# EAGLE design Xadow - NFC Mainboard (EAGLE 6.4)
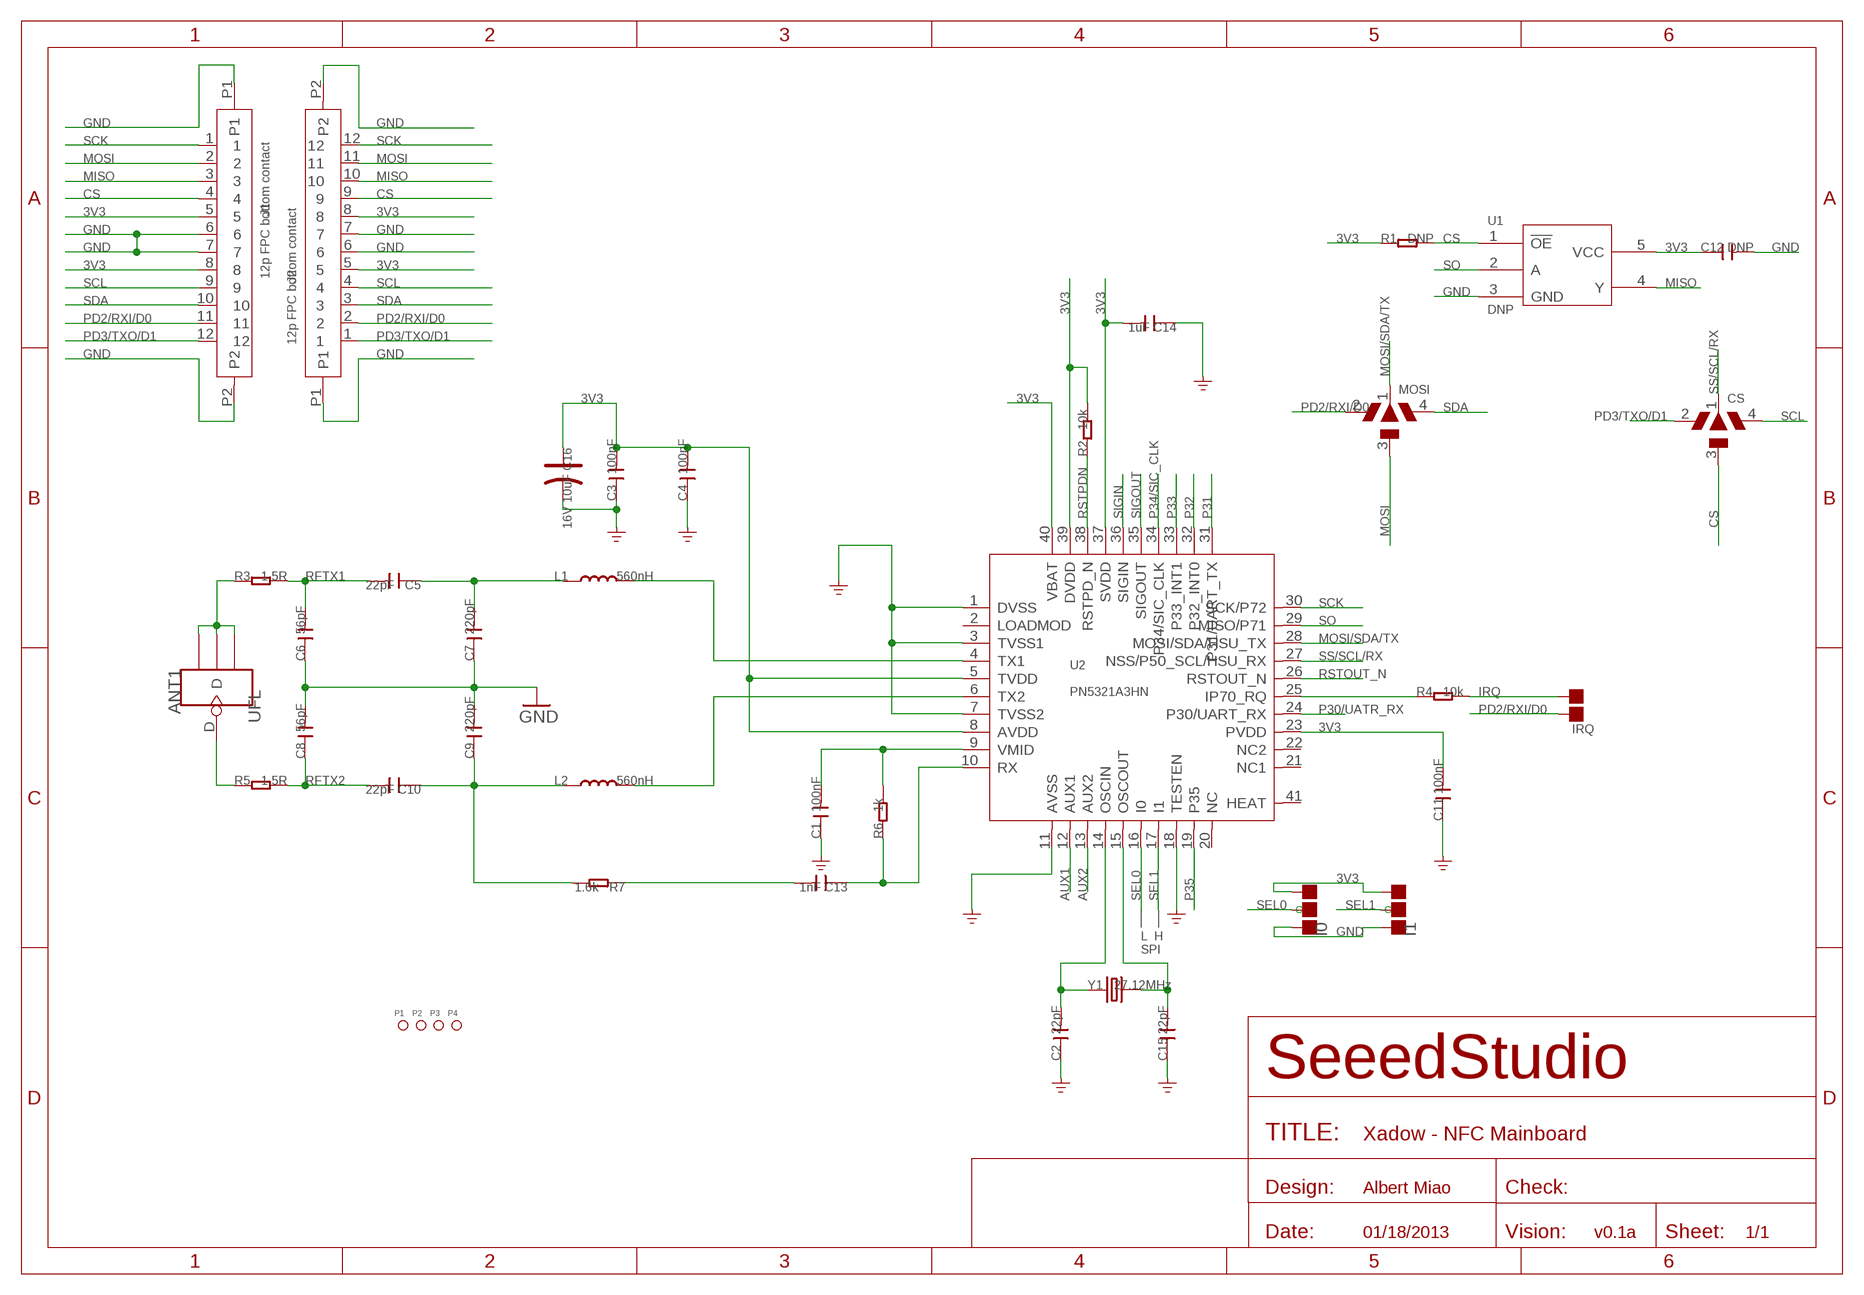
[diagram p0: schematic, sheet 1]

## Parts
ANT1  UFL  ANTENNA-U-FL  [4P-U-FL]
C1  100nF  C-0402  [C0402]
C2  22pF  C-0402  [C0402]
C3  100nF  C-0402  [C0402]
C4  100nF  C-0402  [C0402]
C5  22pF  C-0402  [C0402]
C6  56pF  C-0402  [C0402]
C7  220pF  C-0402  [C0402]
C8  56pF  C-0402  [C0402]
C9  220pF  C-0402  [C0402]
C10  22pF  C-0402  [C0402]
C11  100nF  C-0402  [C0402]
C12  DNP  C-0402  [C0402]
C13  1nF  C-0402  [C0402]
C14  1uF  C-0603  [C0603]
C15  22pF  C-0402  [C0402]
C16  16V 10uF  CAP-AVX-A  [AVX-A]
CS  DNP  PAD-JUMPER-4P  [4P-TRIANGLE]
I0  DNP  PAD-JUMPER-3P-40*40  [3P-SMD-4.1X1.5]
I1  DNP  PAD-JUMPER-3P-40*40  [3P-SMD-4.1X1.5]
IRQ  DNP  PAD-JUMPER-2P  [2P-SMD-1.78X1.27]
J1  12p FPC bottom contact  FPC052002-12LT  [12P-0.5]
J2  12p FPC bottom contact  FPC052002-12LT  [12P-0.5]
L1  560nH  L'0603'  [L0603]
L2  560nH  L'0603'  [L0603]
MOSI  DNP  PAD-JUMPER-4P  [4P-TRIANGLE]
P1  PAD-MARK  [ROUND-MARK-1.0]
P2  PAD-MARK  [ROUND-MARK-1.0]
P3  PAD-MARK  [ROUND-MARK-1.0]
P4  PAD-MARK  [ROUND-MARK-1.0]
R1  DNP  R-0402  [R0402]
R2  10k  R-0402  [R0402]
R3  1.5R  R-0402  [R0402]
R4  10k  R-0402  [R0402]
R5  1.5R  R-0402  [R0402]
R6  1k  R-0402  [R0402]
R7  1.6k  R-0402  [R0402]
U1  DNP  SN74LVC1G125DCKR  [SOT353]
U2  PN5321A3HN  PN532-HVQFN40  [HVQFN40]
Y1  27.12MHz  CRYSTAL'3225'  [4P-SMD-3.2X2.5]

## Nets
3V3: C3.2 C4.2 C11.2 C12.1 C14.2 C16.+ I0.00(L) I1.00(L) J1.5 J1.8 J2.5 J2.8 R1.1 R2.2 U1.5(VCC) U2.5(TVDD) U2.8(AVDD) U2.23(PVDD) U2.37(SVDD) U2.39(DVDD) U2.40(VBAT)
AUX1: U2.12(AUX1)
AUX2: U2.13(AUX2)
CS: CS.3 J1.4 J2.9 R1.2 U1.1(!OE!)
GND: C1.1 C2.1 C3.1 C4.1 C6.1 C7.1 C8.2 C9.2 C11.1 C12.2 C14.1 C15.1 C16.- I0.11(R) I1.11(R) J1.6 J1.7 J1.P1 J1.P2 J2.6 J2.7 J2.P1 J2.P2 U1.3(GND) U2.1(DVSS) U2.3(TVSS1) U2.7(TVSS2) U2.11(AVSS) U2.18(TESTEN)
IRQ: IRQ.1 R4.2
MISO: J1.3 J2.10 U1.4(Y)
MOSI: J1.2 J2.11 MOSI.3
MOSI/SDA/TX: MOSI.1 U2.28(MOSI/SDA/HSU_TX)
N$1: C2.2 U2.14(OSCIN) Y1.2
N$2: C15.2 U2.15(OSCOUT) Y1.4
N$3: L2.2 U2.6(TX2)
N$4: L1.2 U2.4(TX1)
N$5: C5.1 C7.2 L1.1
N$6: C13.2 R7.1
N$7: C9.1 C10.1 L2.1 R7.2
N$9: C1.2 R6.2 U2.9(VMID)
N$11: C13.1 R6.1 U2.10(RX)
N$15: R4.1 U2.25(IP70_RQ)
N$17: ANT1.D R5.1
N$18: ANT1.GND1 ANT1.GND2 ANT1.GND3 R3.1
P30/UATR_RX: U2.24(P30/UART_RX)
P31: U2.31(P31/UART_TX)
P32: U2.32(P32_INT0)
P33: U2.33(P33_INT1)
P34/SIC_CLK: U2.34(P34/SIC_CLK)
P35: U2.19(P35)
PD2/RXI/D0: IRQ.2 J1.11 J2.2 MOSI.2
PD3/TXO/D1: CS.2 J1.12 J2.1
RFTX1: C5.2 C6.2 R3.2
RFTX2: C8.1 C10.2 R5.2
RSTOUT_N: U2.26(RSTOUT_N)
RSTPDN: R2.1 U2.38(RSTPD_N)
SCK: J1.1 J2.12 U2.30(SCK/P72)
SCL: CS.4 J1.9 J2.4
SDA: J1.10 J2.3 MOSI.4
SEL0: I0.MM(C) U2.16(I0)
SEL1: I1.MM(C) U2.17(I1)
SIGIN: U2.36(SIGIN)
SIGOUT: U2.35(SIGOUT)
SO: U1.2(A) U2.29(MISO/P71)
SS/SCL/RX: CS.1 U2.27(NSS/P50_SCL/HSU_RX)
Unconnected: U2.2(LOADMOD) U2.20(NC) U2.21(NC1) U2.22(NC2) U2.41(HEAT)

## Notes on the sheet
- L | H
- SPI
- Albert Miao
- 01/18/2013 | v0.1a

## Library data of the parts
ANT1 = Connector:ANTENNA-U-FL
C1-C15 = Discrete:C*: Ceramic Capacitors
C16 = Discrete:CAP*: Electrolytic Capacitors,Tantalum Capacitors and Super Capacitors
CS MOSI = Discrete:PAD-JUMPER-4P
I0 I1 = Discrete:PAD-JUMPER-3P; PARTNO: DNP
IRQ = Discrete:PAD-JUMPER-2P; PARTNO: DNP
J1 J2 = template:FPC052002-12LT
L1 L2 = Discrete:L*
P1-P4 = Discrete:PAD-MARK; PARTNO: DNP
R1-R7 = Discrete:R*
U1 = Test:SN74LVC1G125DCKR: Signal bus buffer gate
U2 = IC:PN532: NFC Controller http://www.adafruit.com/datasheets/pn532ds.pdf
Y1 = Discrete:CRYSTAL*: CRYSTAL

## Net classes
0 default: width 0.152 mm, drill 0.305 mm, clearance 0.152 mm
1 GND: width 0.152 mm, drill 0.305 mm, clearance 0.152 mm to class 0, clearance 0.152 mm
3 usbvcc: width 0.203 mm, drill 0.305 mm, clearance 0.203 mm

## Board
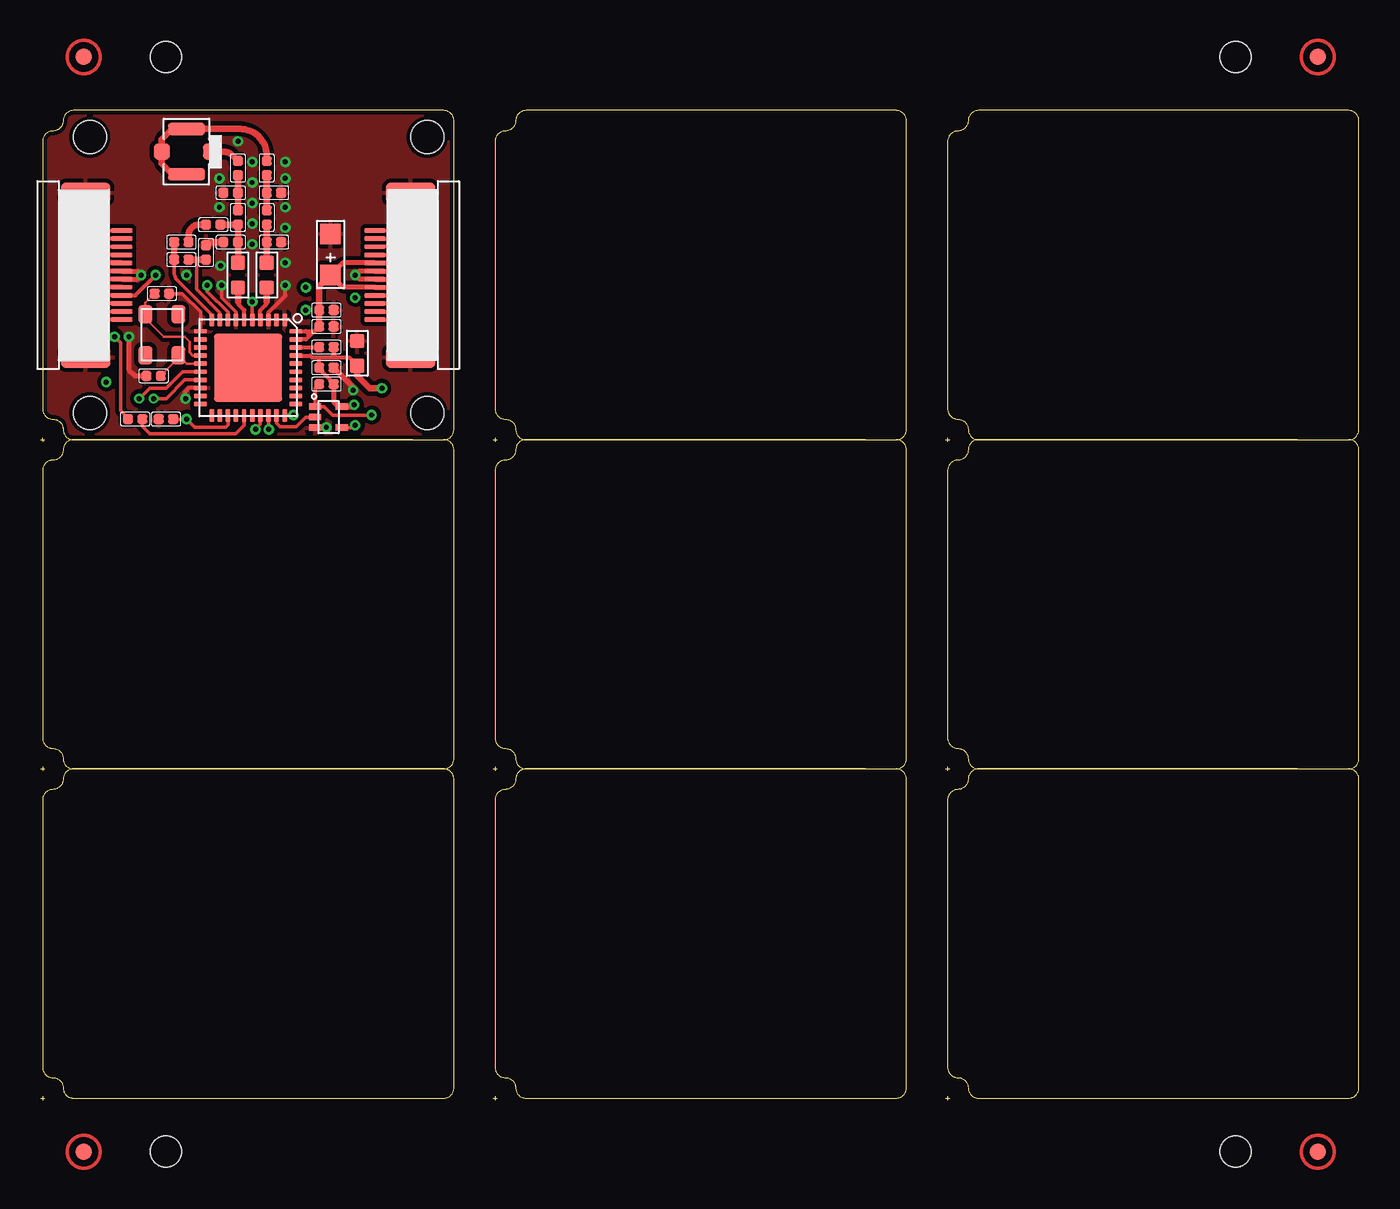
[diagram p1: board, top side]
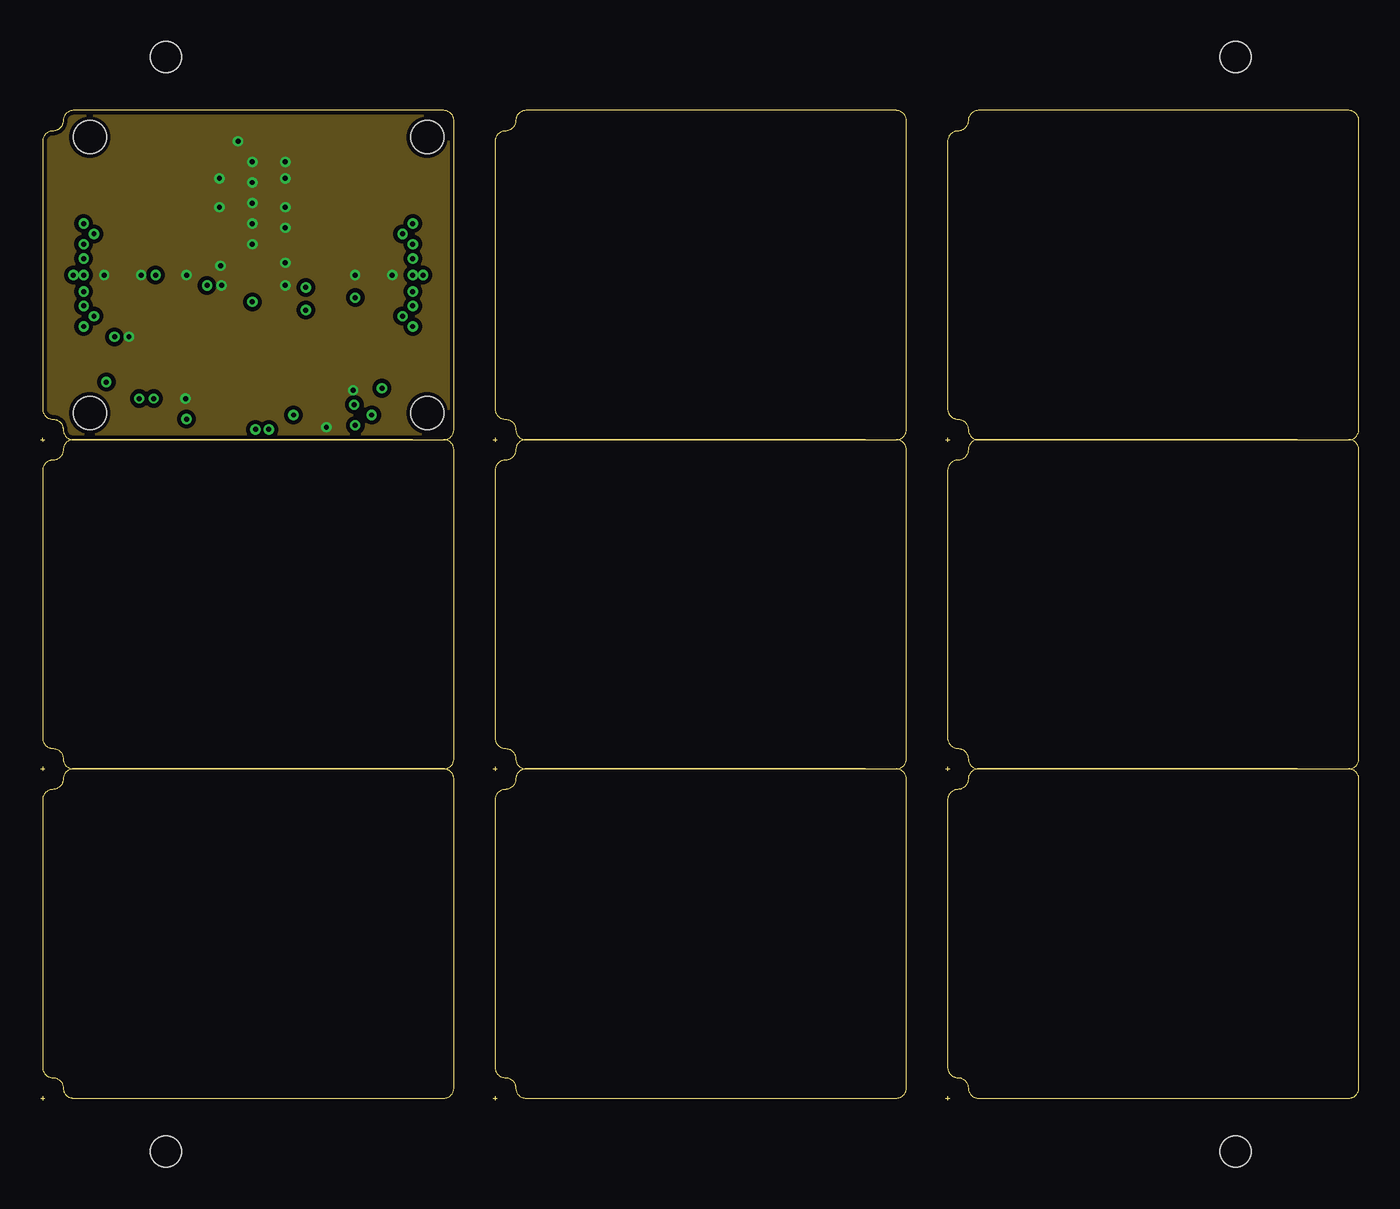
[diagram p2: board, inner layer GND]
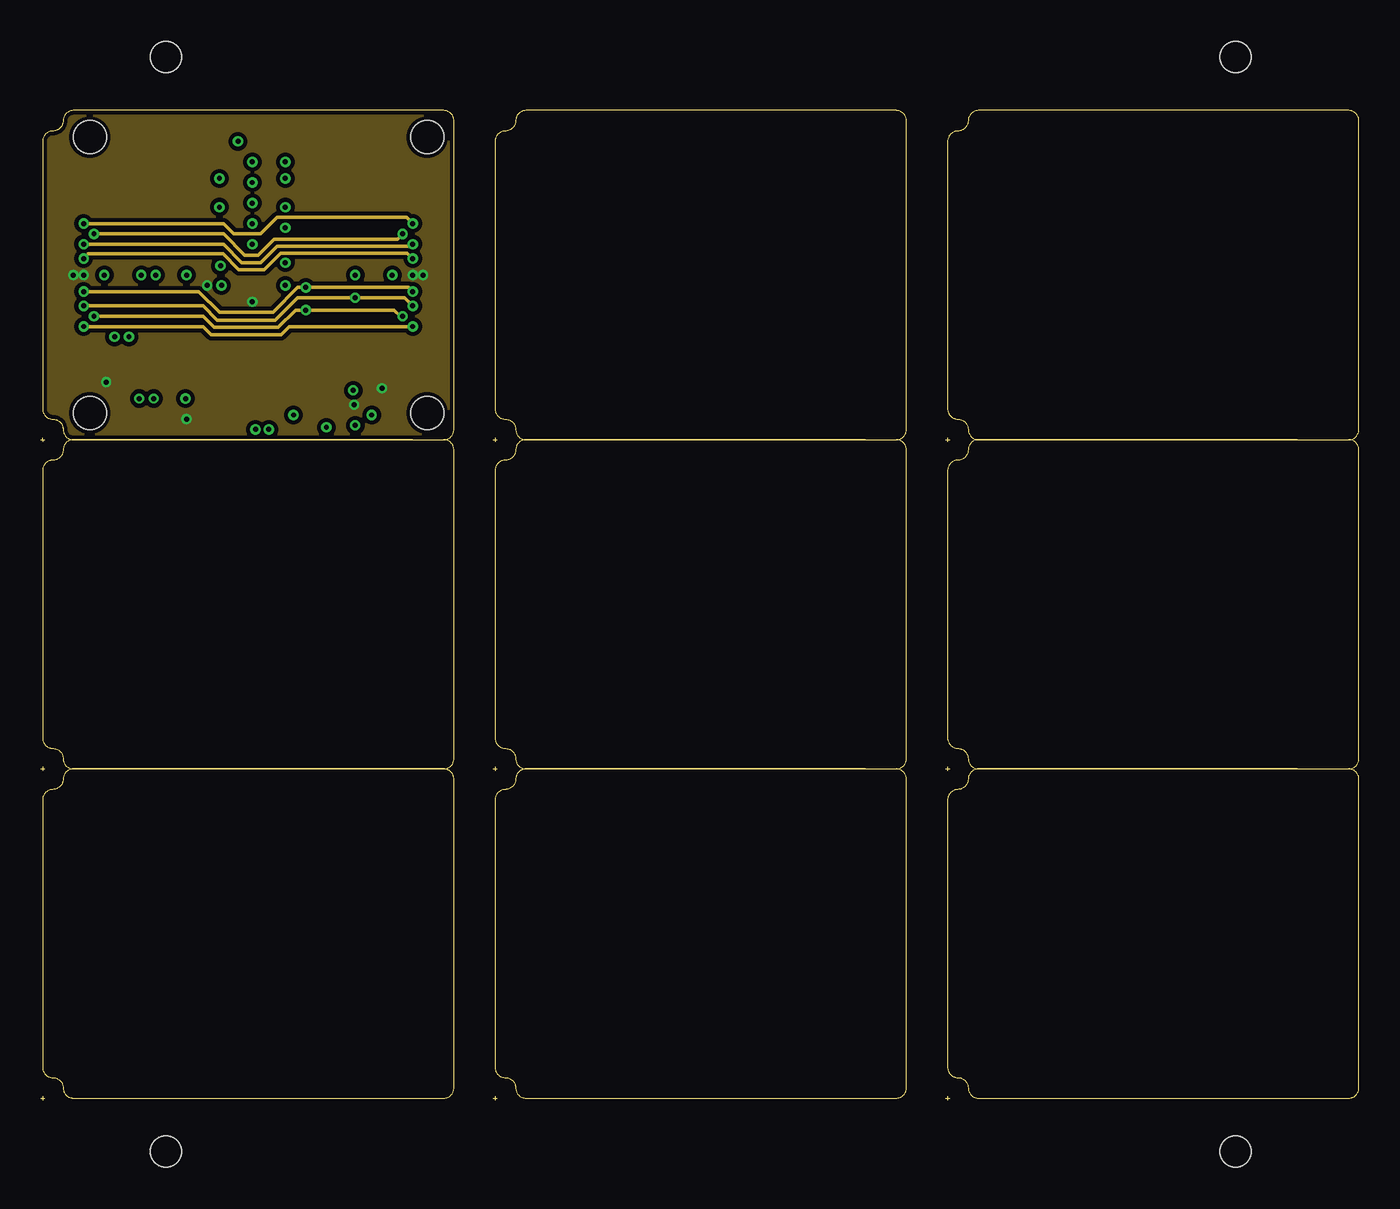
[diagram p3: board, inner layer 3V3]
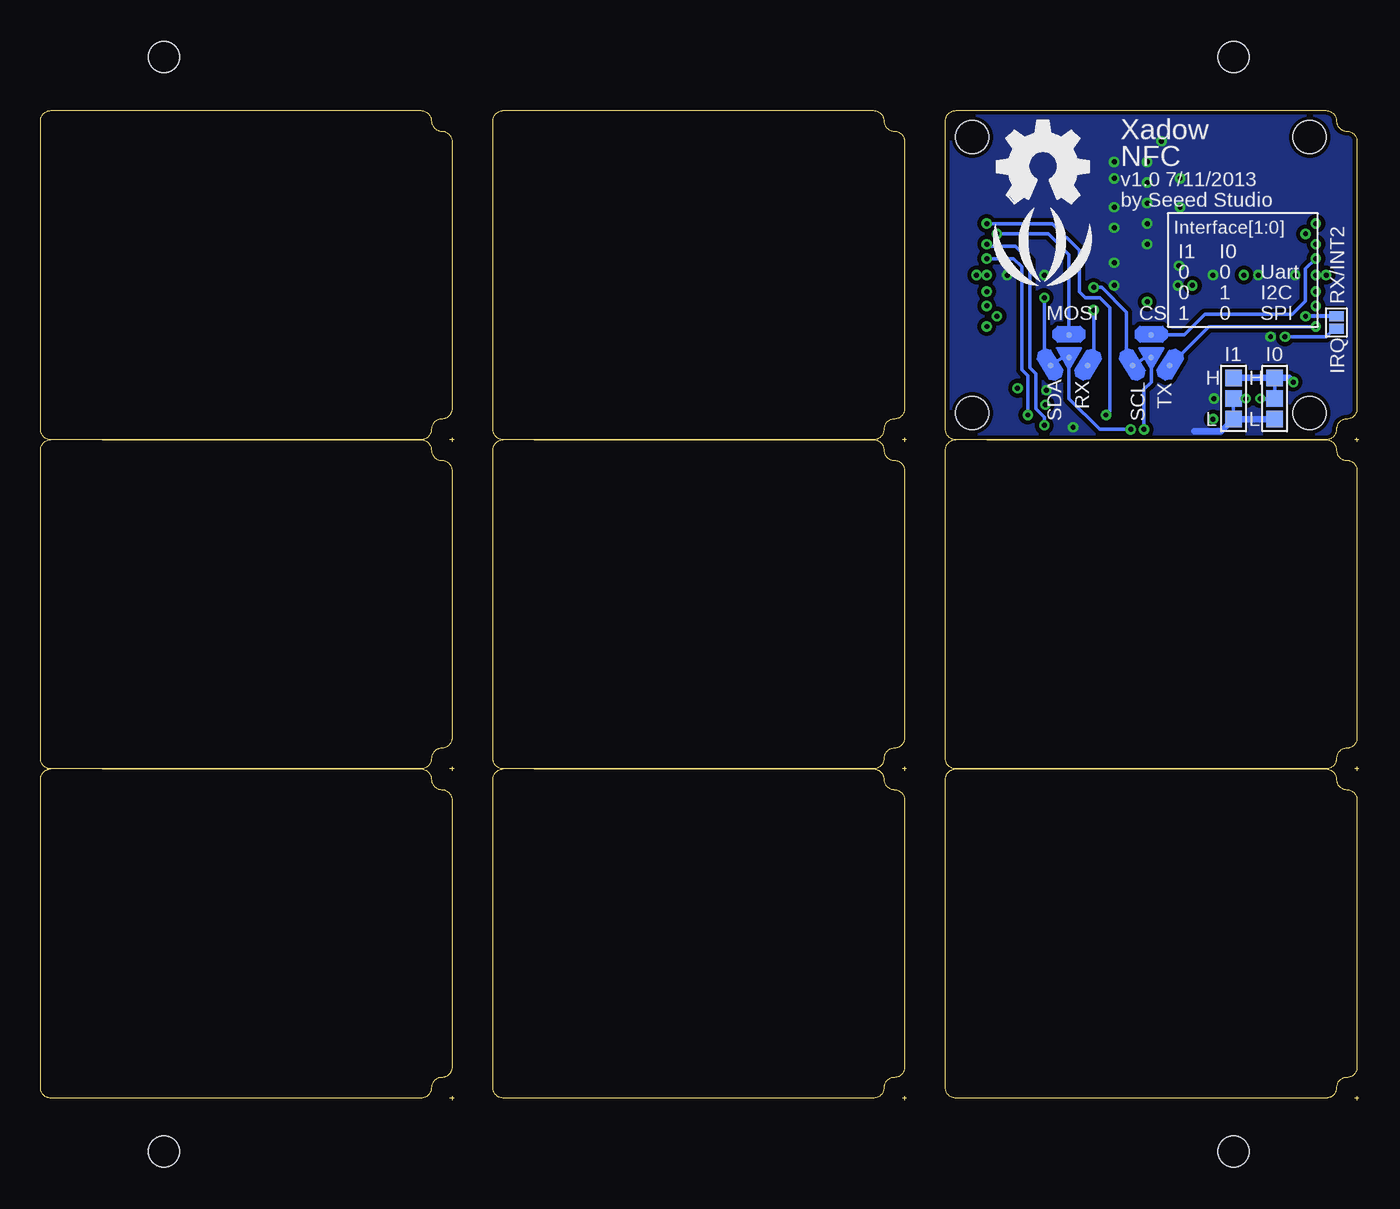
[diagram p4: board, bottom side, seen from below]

Size 81.41 x 61.09 mm. Coordinates in mm from the lower left corner, seen from the top.
Outline: 161 segments
Copper layers (1*2*15*16): Top 0.035mm / dielectric 1.5mm / GND 0.0175mm / dielectric 1.1mm / 3V3 0.0175mm / dielectric 0.2mm / Bottom 0.035mm
Design rules "SeeedStudio_DRU_no_angle_20130527 *": minimum track width 5mil, minimum drill 12mil, track to track 6mil, track to pad 6mil, pad to pad 6mil, via to via 6mil, smd to smd 0mil, copper to edge 10mil, drill to drill 10mil, minimum pad ring 10mil, minimum via ring 6mil, stop-mask expansion 2mil, vias tented up to drill 25mil, thermal gap 10mil
Holes 2.03 mm at 3.05,42.42 3.05,59.44 23.88,59.44 23.88,42.42
Holes 1.91 mm at 73.79,64.39 7.75,64.39 7.75,-3.17 73.79,-3.17
tRestrict: area 4.4,50.7 to 5.7,51.2; area 20,50.7 to 21.3,51.2; 13 lines
bRestrict: 13 lines
Milling: area -16,60.5 to -10.9,61; area -16,59.2 to -10.9,60.4; area -16,58.7 to -10.9,59.1; 24 lines

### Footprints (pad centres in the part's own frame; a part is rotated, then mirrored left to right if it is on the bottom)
4P-U-FL = smd 1.016 x 1.016: D -1.524,0; GND3 1.524,0 | smd 2.286 x 0.762: GND1 0,1.397; GND2 0,-1.397
C0402 = smd 0.635 x 0.635: 1 -0.445,0; 2 0.445,0
C0603 = smd 0.889 x 0.889: 1 -0.762,0; 2 0.762,0
AVX-A = smd 1.27 x 1.27: + -1.27,0; - 1.27,0
4P-TRIANGLE = smd 0.381 x 0.381: 1 0,0; 2 -1.143,0.508; 3 0,-1.397; 4 1.143,0.508
3P-SMD-4.1X1.5 = smd 1.016 x 1.016: 00 -1.27,0; 11 1.27,0; MM 0,0
2P-SMD-1.78X1.27 = smd 0.889 x 0.61: 1 0,0.381; 2 0,-0.381
12P-0.5 = smd 0.3 x 1.3: 1 -2.75,2.35; 2 -2.25,2.35; 3 -1.75,2.35; 4 -1.25,2.35; 5 -0.75,2.35; 6 -0.25,2.35; 7 0.25,2.35; 8 0.75,2.35; 9 1.25,2.35; 10 1.75,2.35; 11 2.25,2.35; 12 2.75,2.35 | smd 1.27 x 3.048: P1 -5.08,0.127; P2 5.08,0.127
L0603 = smd 0.889 x 0.889: 1 -0.762,0; 2 0.762,0
ROUND-MARK-1.0 = smd 1.016 x 1.016: P$1 0,0
R0402 = smd 0.635 x 0.635: 1 -0.445,0; 2 0.445,0
SOT353 = smd 0.4 x 0.75: 1 -0.65,-0.825; 2 0,-0.825; 3 0.65,-0.825; 4 0.65,0.825; 5 -0.65,0.825
HVQFN40 = smd 0.8 x 0.3: 1 -2.95,2.25; 2 -2.95,1.75; 3 -2.95,1.25; 4 -2.95,0.75; 5 -2.95,0.25; 6 -2.95,-0.25; 7 -2.95,-0.75; 8 -2.95,-1.25; 9 -2.95,-1.75; 10 -2.95,-2.25; 21 2.95,-2.25; 22 2.95,-1.75; 23 2.95,-1.25; 24 2.95,-0.75; 25 2.95,-0.25; 26 2.95,0.25; 27 2.95,0.75; 28 2.95,1.25; 29 2.95,1.75; 30 2.95,2.25 | smd 0.3 x 0.8: 11 -2.25,-2.95; 12 -1.75,-2.95; 13 -1.25,-2.95; 14 -0.75,-2.95; 15 -0.25,-2.95; 16 0.25,-2.95; 17 0.75,-2.95; 18 1.25,-2.95; 19 1.75,-2.95; 20 2.25,-2.95; 31 2.25,2.95; 32 1.75,2.95; 33 1.25,2.95; 34 0.75,2.95; 35 0.25,2.95; 36 -0.25,2.95; 37 -0.75,2.95; 38 -1.25,2.95; 39 -1.75,2.95; 40 -2.25,2.95 | smd 4.2 x 4.2: 41 0,0
4P-SMD-3.2X2.5 = smd 1.143 x 0.889: 1 -1.27,1.016; 2 -1.27,-1.016; 3 1.27,-1.016; 4 1.27,1.016

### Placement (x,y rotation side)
ANT1  9.02,58.55 180 top
C1  10.22,52.32 270 top
C2  7.49,49.78 180 top
C3  17.65,47.75 180 top
C4  17.65,48.77 180 top
C5  13.97,54.48 90 top
C6  14.41,56.01 180 top
C7  14.41,52.96 180 top
C8  11.75,56.01 180 top
C9  11.75,52.96 180 top
C10  12.19,54.48 90 top
C11  7.75,42.04 0 top
C12  17.65,45.21 0 top
C13  8.7,52.96 0 top
C14  19.56,46.1 270 top
C15  6.99,44.7 0 top
C16  17.91,52.2 90 top
CS  12.83,45.85 180 bottom
I0  5.21,43.31 270 bottom
I1  7.75,43.31 270 bottom
IRQ  1.4,48.01 180 bottom
J1  2.67,50.93 270 top
J2  22.99,50.93 90 top
L1  13.97,50.93 270 top
L2  12.19,50.93 270 top
MOSI  17.91,45.85 180 bottom
P1  not placed on the board
P2  not placed on the board
P3  not placed on the board
P4  not placed on the board
R1  17.65,44.2 180 top
R2  17.65,46.48 0 top
R3  13.97,57.53 270 top
R4  5.84,42.04 180 top
R5  12.19,57.53 270 top
R6  8.7,51.88 0 top
R7  10.67,54.04 0 top
U1  17.78,42.16 270 top
U2  12.83,45.21 270 top
U$4  [LOGO_SILK]  19.56,51.94 0 bottom
U$5  [OSHW_FILLX200_NOTEXT]  22.35,55.37 0 bottom
Y1  7.49,47.24 270 top

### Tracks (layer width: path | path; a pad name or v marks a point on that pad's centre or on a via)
3V3  (via drill 0.3 pad 0.64)
  Top 0.203: U2.5 v13.08,49.27 v13.08,49.28 | U2.23 11.58,41.68 11.43,41.53 9.53,41.53 v9.02,42.04 C11.2 | U2.8 11.58,48.62 10.29,49.91 v10.29,50.29
  Top 0.254: 16.51,47.09 16.51,47.34 16.38,47.46 | 16.51,47.09 16.38,46.96 U2.39 | U2.40 16.38,47.46 | 16.51,47.09 17.17,47.75 C3.2 16.92,47.46 16.38,47.46 | 18.03,44.32 17.21,45.15 C12.1 17.21,45.72 | U2.37 16.65,45.96 16.76,45.85 17.08,45.85 | 17.08,45.85 17.14,45.85 | 17.14,45.85 17.34,45.85 | 18.1,45.85 18.22,45.85 | 18.22,45.85 19.05,45.85 C14.2 | 17.21,45.72 17.21,45.78 17.14,45.85 | 17.21,45.72 17.08,45.85 | 17.21,45.72 17.34,45.85 | 17.34,45.85 17.97,45.85 | 17.97,45.85 18.1,45.85 | 18.1,45.85 18.1,45.97 | 18.1,45.97 17.97,45.85 | 18.1,45.97 18.22,45.85 | R2.2 18.1,45.97
  Top 0.305: J1.5 3.42,51.68 v2.67,50.93 3.42,50.18 J1.8 | R1.1 18.1,43.12 18.41,42.8 18.59,42.8 | 18.59,42.8 U1.5 | 18.59,42.8 19.24,42.8 v19.37,42.93 | J2.8 22.24,51.68 v22.99,50.93 22.24,50.18 J2.5 18.66,50.18 C16.+ 18.66,51.68 J2.8
  Top 0.406: C3.2 C4.2 17.21,50.23 C16.+ | v21.08,43.94 20.32,43.94 19.56,44.7 C14.2
  Top 0.61: v2.03,50.93 v2.67,50.93 | v22.99,50.93 v23.62,50.93
  Bottom 0.406: I1.00 I0.00 4.32,44.58 v4.06,44.32
  pour 3V3 (isolate 0.254): 0.13,61.09 25.53,61.09 25.53,40.77 0.13,40.77
CS  (via drill 0.3 pad 0.64)
  Top 0.203: v20.45,42.29 18.03,42.29 17.51,42.81 U1.1 16.95,43.94 R1.2
  Top 0.254: J1.4 2.9,52.18 v2.67,51.94 | J2.9 22.75,52.18 v22.99,51.94
  3V3 0.203: v2.67,51.94 2.96,52.23 11.27,52.23 12.23,51.27 13.8,51.27 14.82,52.28 22.64,52.28 v22.99,51.94
  Bottom 0.203: CS.3 10.79,47.24 9.53,48.51 4.12,48.51 3.3,49.33 3.3,51.31 v2.67,51.94 | v20.45,42.29 20.45,44.7 20.83,45.09 20.83,51.44 21.34,51.94 v22.99,51.94
GND  (via drill 0.3 pad 0.64)
  Top 0.203: U2.7 12.08,48.63 11.18,49.53 v11.18,50.29 | U2.11 9.88,48.67 8.76,49.78 C2.1
  Top 0.254: C12.2 18.16,45.21 | U2.3 14.08,48.62 15.11,49.66 v15.11,50.29 | U2.18 9.16,43.96 8.89,43.69 8.89,43.37 v8.95,43.31
  Top 0.305: v19.3,43.81 19.3,44.01 C12.2 | U1.3 17.64,41.51 v17.65,41.53 | v5.46,47.12 5.46,45.09 5.84,44.7 C15.1 | J1.6 4.19,51.18 v3.94,50.93 4.19,50.68 J1.7 5.97,50.68 v6.22,50.93 5.97,51.18 J1.6 | J2.6 21.47,50.68 v21.72,50.93 21.47,51.18 J2.7 19.68,51.18 v19.43,50.93 19.68,50.68 J2.6
  Top 0.406: C9.2 10.41,52.96 C1.1
  Bottom 0.406: I0.11 I1.11 8.51,41.27 10.16,41.27
  other vias: 13.08,52.83 13.08,54.1 13.08,55.37 13.08,56.64 13.08,57.91 12.19,59.18 11.11,51.5 15.11,51.69 15.11,53.85 15.11,55.12 15.11,56.9 15.11,57.91 11.05,55.12 11.05,56.9 9.02,50.93
  pour Top (isolate 0.254): 0.13,61.09 25.53,61.09 25.53,40.77 0.13,40.77
  pour GND (isolate 0.254): 0.13,61.09 25.53,61.09 25.53,40.77 0.13,40.77
  pour Bottom (isolate 0.254): 0.13,61.09 25.53,61.09 25.53,40.77 0.13,40.77
IRQ  (via drill 0.3 pad 0.64)
  Top 0.203: R4.2 5.4,42.1 4.95,42.55 4.95,46.74 v4.57,47.12
  Bottom 0.203: v4.57,47.12 2.03,47.12 1.52,47.62 IRQ.1
MISO  (via drill 0.3 pad 0.64)
  Top 0.203: J1.3 2.82,52.68 v2.67,52.83 | v22.99,52.83 22.86,52.7 20.66,52.7 J2.10 | U1.4 19.29,41.51 v19.43,41.66
  3V3 0.203: v2.67,52.83 11.3,52.83 12.43,51.7 13.6,51.7 14.61,52.7 22.86,52.7 v22.99,52.83
  Bottom 0.203: v22.99,52.83 22.86,52.7 21.21,52.7 20.32,51.82 20.32,45.21 19.94,44.83 19.94,42.67 19.43,42.16 v19.43,41.66
MOSI  (via drill 0.3 pad 0.64)
  Top 0.254: J1.2 3.59,53.18 v3.3,53.47 | J2.11 22.06,53.18 v22.35,53.47
  3V3 0.203: v3.3,53.47 11.3,53.47 12.61,52.16 13.42,52.16 14.41,53.15 22.03,53.15 v22.35,53.47
  Bottom 0.203: MOSI.3 17.91,52.2 19.18,53.47 v22.35,53.47
MOSI/SDA/TX  (via drill 0.3 pad 0.64)
  Top 0.203: U2.28 14.08,41.42 v14.1,41.4
  Bottom 0.203: v14.1,41.4 16,41.4 17.91,43.31 MOSI.1
N$1
  Top 0.152: U2.14 9.41,45.96 9.21,46.16 9.21,46.8 8.89,47.12 7.62,47.12 6.35,48.39 Y1.2 6.48,49.21 C2.2
N$2
  Top 0.152: U2.15 9.02,45.46 Y1.4 8.51,45.78 C15.2
N$3
  Top 0.254: U2.6 12.58,48.76 12.27,49.08 arc-45 12.19,49.25 12.19,49.28
  Top 0.406: 12.19,49.28 L2.2
N$4
  Top 0.254: U2.4 13.58,48.76 13.88,49.06 arc45 13.97,49.28
  Top 0.406: 13.97,49.28 L1.2
N$5
  Top 0.406: L1.1 C7.2 C5.1
N$6
  Top 0.406: R7.1 9.78,54.04 arc90 9.14,53.4 C13.2
N$7
  Top 0.406: L2.1 C9.1 C10.1 R7.2
N$9
  Top 0.203: U2.9 11.08,48.61 9.65,50.04 9.65,51.56 9.65,51.69 | 9.65,51.69 9.65,51.88 | 9.65,51.69 9.53,51.82 | 9.65,51.69 9.78,51.82
  Top 0.406: R6.2 9.65,51.88 C1.2
N$11
  Top 0.203: U2.10 10.58,48.25 arc45 10.42,48.64 8.48,50.58 arc-45 8.25,51.12 R6.1
  Top 0.406: C13.1 R6.1
N$15
  Top 0.203: U2.25 12.58,41.66 12.06,41.15 6.73,41.15 6.29,41.59 R4.1
N$17
  Top 0.406: ANT1.D 11.3,58.55 arc-45 11.84,58.32 R5.1
N$18
  Top 0.406: ANT1.GND1 8.13,57.15 7.49,57.78 ANT1.GND3 7.49,59.31 8.13,59.94 ANT1.GND2 12.32,59.94 arc-90 13.97,58.29 R3.1
PD2/RXI/D0  (via drill 0.3 pad 0.64)
  Top 0.203: J1.11 3.59,48.68 v3.3,48.39
  Top 0.254: J2.2 22.06,48.68 v22.35,48.39
  3V3 0.203: v22.35,48.39 22.23,48.39 21.84,48.77 v16.38,48.77 15.75,48.77 14.68,47.7 10.72,47.7 10.03,48.39 v3.3,48.39
  Bottom 0.203: 16.76,44.58 MOSI.2 16.76,45.59 16.38,45.97 v16.38,48.77
  Bottom 0.254: IRQ.2 v3.3,48.39
PD3/TXO/D1  (via drill 0.3 pad 0.64)
  Top 0.254: v2.67,47.75 3.68,47.75 4.11,48.18 J1.12 | v22.99,47.75 21.97,47.75 21.55,48.18 J2.1
  3V3 0.203: v2.67,47.75 10.03,47.75 10.54,47.24 14.86,47.24 15.37,47.75 v22.99,47.75
  Bottom 0.203: v2.67,47.75 9.27,47.75 CS.2
RFTX1
  Top 0.406: C5.2 C6.2 R3.2
RFTX2
  Top 0.406: C10.2 C8.1 R5.2
RSTPDN
  Top 0.254: U2.38 17.19,46.46 R2.1
SCK  (via drill 0.3 pad 0.64)
  Top 0.203: U2.30 15.59,42.26 v15.62,42.29 | v22.99,54.1 22.1,54.1 21.67,53.68 J2.12 | J1.1 4.11,53.68 3.68,54.1 v2.67,54.1
  3V3 0.203: v2.67,54.1 11.3,54.1 11.94,53.47 13.59,53.47 14.61,54.48 22.61,54.48 v22.99,54.1
  Bottom 0.203: v15.62,42.29 15.38,42.54 15.38,48.9 16,49.53 16.89,49.53 17.27,49.91 17.27,52.45 18.92,54.1 v22.99,54.1
SCL  (via drill 0.3 pad 0.64)
  Top 0.254: v2.67,49.91 2.9,49.68 J1.9 5.86,49.68 v7.11,50.93 | J2.4 22.75,49.68 v22.99,49.91
  3V3 0.203: v2.67,49.91 9.78,49.91 11.05,48.64 14.35,48.64 15.88,50.16 v16.38,50.16 22.73,50.16 v22.99,49.91
  Bottom 0.203: v16.38,50.16 15.88,50.16 14.35,48.64 14.35,46.35 13.97,45.97 CS.4 12.83,46.1
SDA  (via drill 0.3 pad 0.64)
  Top 0.254: J1.10 2.82,49.18 v2.67,49.02 | J2.3 22.83,49.18 v22.99,49.02
  3V3 0.203: v2.67,49.02 10.03,49.02 10.9,48.15 14.5,48.15 15.88,49.53 v19.43,49.53 22.48,49.53 v22.99,49.02
  Bottom 0.203: 19.43,49.02 v19.43,49.53 19.43,46.35 19.05,45.97 MOSI.4 17.91,46.1
SEL0  (via drill 0.3)
  Top 0.203: U2.16 8.77,44.96 7.75,43.94 6.73,43.94 v6.1,43.31
  Bottom 0.203: I0.MM 5.21,44.58
  Bottom 0.254: v6.1,43.31 I0.MM
SEL1  (via drill 0.3)
  Top 0.203: U2.17 8.9,44.46 I1.MM v6.99,43.31
  Bottom 0.203: I1.MM 7.75,42.04
  Bottom 0.254: v6.99,43.31 I1.MM
SO
  Top 0.203: U2.29 14.58,41.78 14.78,41.58 15.8,41.58 16.38,42.16 U1.2 17.14,42.16
SS/SCL/RX  (via drill 0.3 pad 0.64)
  Top 0.203: U2.27 13.58,41.71 v13.27,41.4
  Bottom 0.203: CS.1 12.83,44.32 13.27,43.88 v13.27,41.4
(copper drawn outside any net)
  shapes: 3V3 area x1, Bottom area x1, GND area x1, Top area x1

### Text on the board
Top: Top Layer : 1Oz/0.035mm
GND: Layer 2 : 0.5Oz/0.0175mm
3V3: Layer 3 : 0.5Oz/0.0175mm
Bottom: Bottom Layer : 1Oz/0.035mm
bPlace: Xadow | NFC | v1.0 7/11/2013 | by Seeed Studio | Interface[1:0] | I0 | I1 | Uart | 0 | 0 | RX/INT2 | I2C | 1 | 0 | SPI | 0 | 1 | IRQ | H | H | TX | RX | L | L | SCL | SDA
Milling: 0.2mm | PCB(FR-4) Stack: | 0.295mm | 0.8mm | 0.2mm
tDocu: J1 | J2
